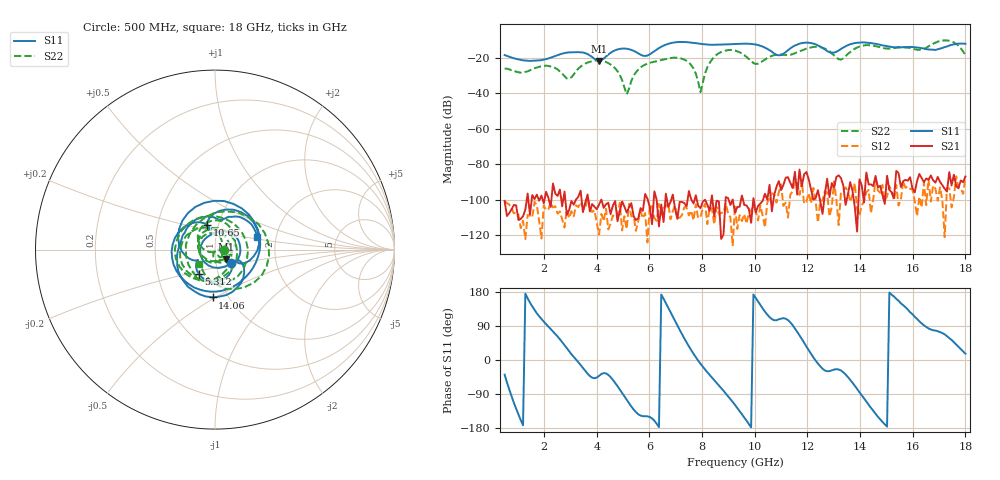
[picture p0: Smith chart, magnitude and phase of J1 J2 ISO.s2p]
!Agilent Technologies,N5230A,MY45001360,A.07.50.67
!Agilent N5230A: A.07.50.67
!Date: Tuesday, April 16, 2024 17:33:52
!Correction: S11(Full 2 Port(1,2))
!S21(Full 2 Port(1,2))
!S12(Full 2 Port(1,2))
!S22(Full 2 Port(1,2))
!S2P File: Measurements: S11, S21, S12, S22:
# Hz S  dB  R 50
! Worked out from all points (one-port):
!   201 points, 500 MHz to 18 GHz, reference 50 ohm
!   lowest |S11| = -21.9 dB at 4.088 GHz (marker M1), VSWR 1.17, Z = 56 - j6.03 ohm
!   |S11| at or under -10 dB: start of sweep to end of sweep
!   S11 on the Smith chart (normalised r, x): 500 MHz: 1.19, -0.18; 5.312 GHz: 0.81, -0.23; 10.65 GHz: 0.88, +0.25; 14.06 GHz: 0.85, -0.49; 18 GHz: 1.59, +0.24
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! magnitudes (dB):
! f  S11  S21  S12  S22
! 500 MHz  -18.6  -100.7  -100.9  -26.2
! 2.163 GHz  -20.5  -99.0  -105.4  -24.8
! 2.95 GHz  -17.1  -105.8  -110.3  -31.9
! 3.475 GHz  -17.2  -107.0  -104.4  -24.2
! 4.088 GHz  -21.9  -102.8  -119.7  -21.6
! 4.787 GHz  -15.4  -112.1  -109.7  -27.7
! 5.138 GHz  -15.0  -107.3  -116.5  -40.7
! 5.312 GHz  -15.7  -102.0  -109.3  -33.2
! 6.362 GHz  -14.6  -115.1  -102.4  -21.7
! 7.412 GHz  -11.3  -103.8  -104.6  -21.9
! 7.763 GHz  -11.9  -97.5  -102.6  -29.0
! 7.938 GHz  -12.3  -104.8  -109.7  -39.5
! 8.375 GHz  -12.8  -97.6  -105.2  -21.1
! 9.25 GHz  -12.4  -107.3  -103.3  -16.1
! 10.04 GHz  -12.7  -107.3  -106.1  -23.6
! 10.65 GHz  -16.7  -106.5  -96.5  -19.1
! 12.22 GHz  -12.1  -99.9  -93.4  -14.0
! 13.28 GHz  -15.1  -87.8  -95.9  -21.2
! 14.06 GHz  -11.5  -92.0  -103.2  -13.4
! 15.11 GHz  -13.8  -94.5  -92.4  -14.9
! 17.3 GHz  -13.8  -95.4  -93.4  -10.4
! 18 GHz  -12.2  -87.0  -87.5  -18.7
